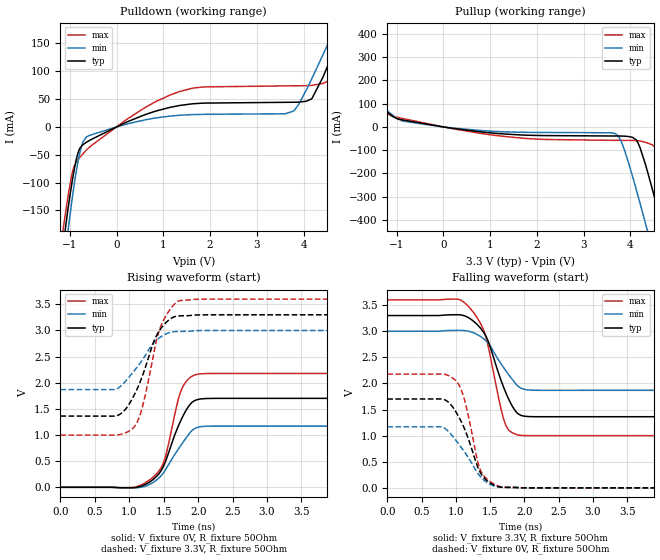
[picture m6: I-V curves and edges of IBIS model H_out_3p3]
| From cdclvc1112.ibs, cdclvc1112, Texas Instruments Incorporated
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|   H_out_3p3
[Model]   H_out_3p3
|Signals :   Y0, Y1, Y2, Y3, Y4, Y5, Y6, Y7, Y8 and Y9
Model_type   Output
Polarity   Non-Inverting
Enable   Active-Low
Vmeas   = 1.62
Vref   = 1.65
Cref   = 2pF
Rref   = 50
|   typ   min   max
C_comp   504.2f   303.5f   628.8f
|C_comp (High state)   59.85f   45.44f   79.75f
[Voltage Range]   3.3   3   3.6
[Temperature Range]   25   85   -40
[Pullup Reference]   3.3   3   3.6
[Pulldown Reference]   0   0   0
[Power Clamp Reference]   3.3   3   3.6
[GND Clamp Reference]   0   0   0
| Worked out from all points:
|   slope of the pulldown table from 0 to 0.495 V, typ, clamps not added: 27.2 ohm
|   slope of the pullup table from 0 to 0.495 V, typ, clamps not added: 36.2 ohm
|   falling waveform, V_fixture 3.3V, R_fixture 50Ohm: 20-80 % time 317ps typ, 343ps min, 272ps max; typ from 3.3 V to 1.36 V
|   rising waveform, V_fixture 0V, R_fixture 50Ohm: 20-80 % time 307ps typ, 350ps min, 240ps max; typ from 0 V to 1.7 V
|   rising waveform, V_fixture 3.3V, R_fixture 50Ohm: 20-80 % time 334ps typ, 376ps min, 271ps max; typ from 1.36 V to 3.3 V
|   falling waveform, V_fixture 0V, R_fixture 50Ohm: 20-80 % time 297ps typ, 360ps min, 219ps max; typ from 1.7 V to 0 V
[Pulldown]
|   Voltage   I(typ)   I(min)   I(max)
-3.3V     -1.958A    -1.947A    -1.97A
-1.176V   -239.8mA   -284.2mA   -204.4mA
-1.048V   -153.1mA   -193.4mA   -130mA
-834.9mV  -49.72mA   -67.1mA    -59.94mA
-627mV    -26.68mA   -17.28mA   -40.09mA
1.338V    38.4mA     20.94mA    63.33mA
3.61V     44.25mA    23.67mA    73.76mA
4.184V    51.58mA    87.88mA    74.74mA
4.769V    161.9mA    195.1mA    121.8mA
4.966V    204.2mA    232.5mA    168.3mA
5.244V    264.6mA    285.4mA    236.7mA
6.6V      574.1mA    552mA      595.4mA
[Pullup]
|   Voltage   I(typ)   I(min)   I(max)
-3.3V     508.4mA    459.9mA    557.7mA
-884.4mV  30.32mA    25.99mA    36.8mA
1.224V    -29.31mA   -20.47mA   -39.27mA
3.675V    -39.06mA   -28.42mA   -57.69mA
3.838V    -39.47mA   -79.81mA   -57.84mA
4.041V    -44.36mA   -209.4mA   -58.07mA
4.17V     -71.59mA   -301.6mA   -59.41mA
4.368V    -193.5mA   -448.9mA   -69.29mA
4.531V    -314.7mA   -573.3mA   -89.27mA
4.679V    -429.4mA   -687.7mA   -169.6mA
5.006V    -688.9mA   -942.8mA   -423.5mA
6.6V      -2.002A    -2.217A    -1.777A
[Ramp]
R_load = 50
|   typ   min   max
dV/dt_r   1.02103/3.06956e-010  0.701667/3.50029e-010   1.30718/2.39683e-010
dV/dt_f   1.16244/3.17462e-010  0.678552/3.42443e-010   1.56004/2.72268e-010
[Falling Waveform]
V_fixture = 3.3V
V_fixture_min = 3V
V_fixture_max = 3.6V
R_fixture = 50Ohm
C_fixture = 0F
|   Time   V(typ)   V(min)   V(max)
0s        3.3V       3V         3.6V
1.012ns   3.316V     3.017V     3.615V
1.177ns   3.264V     3.003V     3.481V
1.335ns   3.094V     2.919V     3.205V
1.432ns   2.917V     2.824V     2.913V
1.643ns   2.118V     2.407V     1.603V
1.717ns   1.856V     2.262V     1.232V
1.883ns   1.449V     1.978V     1.022V
2.123ns   1.363V     1.87V      1V
6.248ns   1.363V     1.869V     999.9mV
[Rising Waveform]
V_fixture = 0V
V_fixture_min = 0V
V_fixture_max = 0V
R_fixture = 50Ohm
C_fixture = 0F
|   Time   V(typ)   V(min)   V(max)
0s        3.755nV    5.439nV    2.909nV
1.043ns   -7.92mV    -10.72mV   -3.636mV
1.335ns   137.9mV    84.06mV    181.9mV
1.44ns    276.6mV    190.2mV    329.6mV
1.508ns   434.3mV    299.1mV    512mV
1.695ns   1.118V     696.1mV    1.595V
1.763ns   1.317V     826.6mV    1.881V
1.875ns   1.573V     1.034V     2.091V
1.965ns   1.667V     1.133V     2.155V
6.248ns   1.702V     1.169V     2.179V
[Rising Waveform]
V_fixture = 3.3V
V_fixture_min = 3V
V_fixture_max = 3.6V
R_fixture = 50Ohm
C_fixture = 0F
|   Time   V(typ)   V(min)   V(max)
0s        1.363V     1.869V     999.9mV
817.5ps   1.37V      1.883V     1V
945ps     1.494V     2.028V     1.043V
1.065ns   1.75V      2.218V     1.146V
1.192ns   2.138V     2.441V     1.55V
1.35ns    2.768V     2.753V     2.522V
1.44ns    3.003V     2.862V     3.017V
1.575ns   3.201V     2.957V     3.37V
1.725ns   3.28V      2.982V     3.569V
6.248ns   3.3V       3V         3.6V
[Falling Waveform]
|Gnd
V_fixture = 0V
V_fixture_min = 0V
V_fixture_max = 0V
R_fixture = 50Ohm
C_fixture = 0F
|   Time   V(typ)   V(min)   V(max)
0s        1.702V     1.169V     2.179V
787.5ps   1.703V     1.168V     2.181V
990ps     1.476V     927.2mV    2.062V
1.057ns   1.321V     811mV      1.94V
1.117ns   1.157V     703.7mV    1.722V
1.312ns   420.2mV    291.7mV    532.9mV
1.357ns   291.4mV    214.6mV    340.9mV
1.47ns    119.8mV    88.2mV     149mV
1.657ns   13.73mV    13.9mV     18.48mV
6.248ns   3.755nV    5.439nV    2.909nV
